DATA_BLOCK "IMAC_MOTOR3_I/O"
TITLE =
AUTHOR : Hottendo
FAMILY : IMAC
VERSION : 0.1


  STRUCT
   MOTOR3_001_ACOM : WORD ;	//MOTOR3 - Instance 001 : 'AUTO' Mode  Command Interface
   MOTOR3_001_STAT : WORD ;	//                        'AUTO' Mode  Status Interface
   MOTOR3_001_OSSTAT : WORD ;	//                        OS Status Word
   MOTOR3_001_OSALARM : WORD ;	//                        OS Alarm Word
   MOTOR3_001_OSCOM : WORD ;	//                        OS Command Interface
   MOTOR3_002_ACOM : WORD ;	//MOTOR3 - Instance 002 : 'AUTO' Mode  Command Interface
   MOTOR3_002_STAT : WORD ;	//                        'AUTO' Mode  Status Interface
   MOTOR3_002_OSSTAT : WORD ;	//                        OS Status Word
   MOTOR3_002_OSALARM : WORD ;	//                        OS Alarm Word
   MOTOR3_002_OSCOM : WORD ;	//                        OS Command Interface
   MOTOR3_003_ACOM : WORD ;	//MOTOR3 - Instance 003 : 'AUTO' Mode  Command Interface
   MOTOR3_003_STAT : WORD ;	//                        'AUTO' Mode  Status Interface
   MOTOR3_003_OSSTAT : WORD ;	//                        OS Status Word
   MOTOR3_003_OSALARM : WORD ;	//                        OS Alarm Word
   MOTOR3_003_OSCOM : WORD ;	//                        OS Command Interface
   MOTOR3_004_ACOM : WORD ;	//MOTOR3 - Instance 004 : 'AUTO' Mode  Command Interface
   MOTOR3_004_STAT : WORD ;	//                        'AUTO' Mode  Status Interface
   MOTOR3_004_OSSTAT : WORD ;	//                        OS Status Word
   MOTOR3_004_OSALARM : WORD ;	//                        OS Alarm Word
   MOTOR3_004_OSCOM : WORD ;	//                        OS Command Interface
   MOTOR3_005_ACOM : WORD ;	//MOTOR3 - Instance 005 : 'AUTO' Mode  Command Interface
   MOTOR3_005_STAT : WORD ;	//                        'AUTO' Mode  Status Interface
   MOTOR3_005_OSSTAT : WORD ;	//                        OS Status Word
   MOTOR3_005_OSALARM : WORD ;	//                        OS Alarm Word
   MOTOR3_005_OSCOM : WORD ;	//                        OS Command Interface
   MOTOR3_006_ACOM : WORD ;	//MOTOR3 - Instance 006 : 'AUTO' Mode  Command Interface
   MOTOR3_006_STAT : WORD ;	//                        'AUTO' Mode  Status Interface
   MOTOR3_006_OSSTAT : WORD ;	//                        OS Status Word
   MOTOR3_006_OSALARM : WORD ;	//                        OS Alarm Word
   MOTOR3_006_OSCOM : WORD ;	//                        OS Command Interface
   MOTOR3_007_ACOM : WORD ;	//MOTOR3 - Instance 007 : 'AUTO' Mode  Command Interface
   MOTOR3_007_STAT : WORD ;	//                        'AUTO' Mode  Status Interface
   MOTOR3_007_OSSTAT : WORD ;	//                        OS Status Word
   MOTOR3_007_OSALARM : WORD ;	//                        OS Alarm Word
   MOTOR3_007_OSCOM : WORD ;	//                        OS Command Interface
   MOTOR3_008_ACOM : WORD ;	//MOTOR3 - Instance 008 : 'AUTO' Mode  Command Interface
   MOTOR3_008_STAT : WORD ;	//                        'AUTO' Mode  Status Interface
   MOTOR3_008_OSSTAT : WORD ;	//                        OS Status Word
   MOTOR3_008_OSALARM : WORD ;	//                        OS Alarm Word
   MOTOR3_008_OSCOM : WORD ;	//                        OS Command Interface
   MOTOR3_009_ACOM : WORD ;	//MOTOR3 - Instance 009 : 'AUTO' Mode  Command Interface
   MOTOR3_009_STAT : WORD ;	//                        'AUTO' Mode  Status Interface
   MOTOR3_009_OSSTAT : WORD ;	//                        OS Status Word
   MOTOR3_009_OSALARM : WORD ;	//                        OS Alarm Word
   MOTOR3_009_OSCOM : WORD ;	//                        OS Command Interface
   MOTOR3_010_ACOM : WORD ;	//MOTOR3 - Instance 010 : 'AUTO' Mode  Command Interface
   MOTOR3_010_STAT : WORD ;	//                        'AUTO' Mode  Status Interface
   MOTOR3_010_OSSTAT : WORD ;	//                        OS Status Word
   MOTOR3_010_OSALARM : WORD ;	//                        OS Alarm Word
   MOTOR3_010_OSCOM : WORD ;	//                        OS Command Interface
   MOTOR3_011_ACOM : WORD ;	//MOTOR3 - Instance 011 : 'AUTO' Mode  Command Interface
   MOTOR3_011_STAT : WORD ;	//                        'AUTO' Mode  Status Interface
   MOTOR3_011_OSSTAT : WORD ;	//                        OS Status Word
   MOTOR3_011_OSALARM : WORD ;	//                        OS Alarm Word
   MOTOR3_011_OSCOM : WORD ;	//                        OS Command Interface
   MOTOR3_012_ACOM : WORD ;	//MOTOR3 - Instance 012 : 'AUTO' Mode  Command Interface
   MOTOR3_012_STAT : WORD ;	//                        'AUTO' Mode  Status Interface
   MOTOR3_012_OSSTAT : WORD ;	//                        OS Status Word
   MOTOR3_012_OSALARM : WORD ;	//                        OS Alarm Word
   MOTOR3_012_OSCOM : WORD ;	//                        OS Command Interface
   MOTOR3_013_ACOM : WORD ;	//MOTOR3 - Instance 013 : 'AUTO' Mode  Command Interface
   MOTOR3_013_STAT : WORD ;	//                        'AUTO' Mode  Status Interface
   MOTOR3_013_OSSTAT : WORD ;	//                        OS Status Word
   MOTOR3_013_OSALARM : WORD ;	//                        OS Alarm Word
   MOTOR3_013_OSCOM : WORD ;	//                        OS Command Interface
   MOTOR3_014_ACOM : WORD ;	//MOTOR3 - Instance 014 : 'AUTO' Mode  Command Interface
   MOTOR3_014_STAT : WORD ;	//                        'AUTO' Mode  Status Interface
   MOTOR3_014_OSSTAT : WORD ;	//                        OS Status Word
   MOTOR3_014_OSALARM : WORD ;	//                        OS Alarm Word
   MOTOR3_014_OSCOM : WORD ;	//                        OS Command Interface
   MOTOR3_015_ACOM : WORD ;	//MOTOR3 - Instance 015 : 'AUTO' Mode  Command Interface
   MOTOR3_015_STAT : WORD ;	//                        'AUTO' Mode  Status Interface
   MOTOR3_015_OSSTAT : WORD ;	//                        OS Status Word
   MOTOR3_015_OSALARM : WORD ;	//                        OS Alarm Word
   MOTOR3_015_OSCOM : WORD ;	//                        OS Command Interface
   MOTOR3_016_ACOM : WORD ;	//MOTOR3 - Instance 016 : 'AUTO' Mode  Command Interface
   MOTOR3_016_STAT : WORD ;	//                        'AUTO' Mode  Status Interface
   MOTOR3_016_OSSTAT : WORD ;	//                        OS Status Word
   MOTOR3_016_OSALARM : WORD ;	//                        OS Alarm Word
   MOTOR3_016_OSCOM : WORD ;	//                        OS Command Interface
   MOTOR3_017_ACOM : WORD ;	//MOTOR3 - Instance 017 : 'AUTO' Mode  Command Interface
   MOTOR3_017_STAT : WORD ;	//                        'AUTO' Mode  Status Interface
   MOTOR3_017_OSSTAT : WORD ;	//                        OS Status Word
   MOTOR3_017_OSALARM : WORD ;	//                        OS Alarm Word
   MOTOR3_017_OSCOM : WORD ;	//                        OS Command Interface
   MOTOR3_018_ACOM : WORD ;	//MOTOR3 - Instance 018 : 'AUTO' Mode  Command Interface
   MOTOR3_018_STAT : WORD ;	//                        'AUTO' Mode  Status Interface
   MOTOR3_018_OSSTAT : WORD ;	//                        OS Status Word
   MOTOR3_018_OSALARM : WORD ;	//                        OS Alarm Word
   MOTOR3_018_OSCOM : WORD ;	//                        OS Command Interface
   MOTOR3_019_ACOM : WORD ;	//MOTOR3 - Instance 019 : 'AUTO' Mode  Command Interface
   MOTOR3_019_STAT : WORD ;	//                        'AUTO' Mode  Status Interface
   MOTOR3_019_OSSTAT : WORD ;	//                        OS Status Word
   MOTOR3_019_OSALARM : WORD ;	//                        OS Alarm Word
   MOTOR3_019_OSCOM : WORD ;	//                        OS Command Interface
   MOTOR3_020_ACOM : WORD ;	//MOTOR3 - Instance 020 : 'AUTO' Mode  Command Interface
   MOTOR3_020_STAT : WORD ;	//                        'AUTO' Mode  Status Interface
   MOTOR3_020_OSSTAT : WORD ;	//                        OS Status Word
   MOTOR3_020_OSALARM : WORD ;	//                        OS Alarm Word
   MOTOR3_020_OSCOM : WORD ;	//                        OS Command Interface
   MOTOR3_021_ACOM : WORD ;	//MOTOR3 - Instance 021 : 'AUTO' Mode  Command Interface
   MOTOR3_021_STAT : WORD ;	//                        'AUTO' Mode  Status Interface
   MOTOR3_021_OSSTAT : WORD ;	//                        OS Status Word
   MOTOR3_021_OSALARM : WORD ;	//                        OS Alarm Word
   MOTOR3_021_OSCOM : WORD ;	//                        OS Command Interface
   MOTOR3_022_ACOM : WORD ;	//MOTOR3 - Instance 022 : 'AUTO' Mode  Command Interface
   MOTOR3_022_STAT : WORD ;	//                        'AUTO' Mode  Status Interface
   MOTOR3_022_OSSTAT : WORD ;	//                        OS Status Word
   MOTOR3_022_OSALARM : WORD ;	//                        OS Alarm Word
   MOTOR3_022_OSCOM : WORD ;	//                        OS Command Interface
   MOTOR3_023_ACOM : WORD ;	//MOTOR3 - Instance 023 : 'AUTO' Mode  Command Interface
   MOTOR3_023_STAT : WORD ;	//                        'AUTO' Mode  Status Interface
   MOTOR3_023_OSSTAT : WORD ;	//                        OS Status Word
   MOTOR3_023_OSALARM : WORD ;	//                        OS Alarm Word
   MOTOR3_023_OSCOM : WORD ;	//                        OS Command Interface
   MOTOR3_024_ACOM : WORD ;	//MOTOR3 - Instance 024 : 'AUTO' Mode  Command Interface
   MOTOR3_024_STAT : WORD ;	//                        'AUTO' Mode  Status Interface
   MOTOR3_024_OSSTAT : WORD ;	//                        OS Status Word
   MOTOR3_024_OSALARM : WORD ;	//                        OS Alarm Word
   MOTOR3_024_OSCOM : WORD ;	//                        OS Command Interface
   MOTOR3_025_ACOM : WORD ;	//MOTOR3 - Instance 025 : 'AUTO' Mode  Command Interface
   MOTOR3_025_STAT : WORD ;	//                        'AUTO' Mode  Status Interface
   MOTOR3_025_OSSTAT : WORD ;	//                        OS Status Word
   MOTOR3_025_OSALARM : WORD ;	//                        OS Alarm Word
   MOTOR3_025_OSCOM : WORD ;	//                        OS Command Interface
  END_STRUCT ;
BEGIN
   MOTOR3_001_ACOM := W#16#0;
   MOTOR3_001_STAT := W#16#0;
   MOTOR3_001_OSSTAT := W#16#0;
   MOTOR3_001_OSALARM := W#16#0;
   MOTOR3_001_OSCOM := W#16#0;
   MOTOR3_002_ACOM := W#16#0;
   MOTOR3_002_STAT := W#16#0;
   MOTOR3_002_OSSTAT := W#16#0;
   MOTOR3_002_OSALARM := W#16#0;
   MOTOR3_002_OSCOM := W#16#0;
   MOTOR3_003_ACOM := W#16#0;
   MOTOR3_003_STAT := W#16#0;
   MOTOR3_003_OSSTAT := W#16#0;
   MOTOR3_003_OSALARM := W#16#0;
   MOTOR3_003_OSCOM := W#16#0;
   MOTOR3_004_ACOM := W#16#0;
   MOTOR3_004_STAT := W#16#0;
   MOTOR3_004_OSSTAT := W#16#0;
   MOTOR3_004_OSALARM := W#16#0;
   MOTOR3_004_OSCOM := W#16#0;
   MOTOR3_005_ACOM := W#16#0;
   MOTOR3_005_STAT := W#16#0;
   MOTOR3_005_OSSTAT := W#16#0;
   MOTOR3_005_OSALARM := W#16#0;
   MOTOR3_005_OSCOM := W#16#0;
   MOTOR3_006_ACOM := W#16#0;
   MOTOR3_006_STAT := W#16#0;
   MOTOR3_006_OSSTAT := W#16#0;
   MOTOR3_006_OSALARM := W#16#0;
   MOTOR3_006_OSCOM := W#16#0;
   MOTOR3_007_ACOM := W#16#0;
   MOTOR3_007_STAT := W#16#0;
   MOTOR3_007_OSSTAT := W#16#0;
   MOTOR3_007_OSALARM := W#16#0;
   MOTOR3_007_OSCOM := W#16#0;
   MOTOR3_008_ACOM := W#16#0;
   MOTOR3_008_STAT := W#16#0;
   MOTOR3_008_OSSTAT := W#16#0;
   MOTOR3_008_OSALARM := W#16#0;
   MOTOR3_008_OSCOM := W#16#0;
   MOTOR3_009_ACOM := W#16#0;
   MOTOR3_009_STAT := W#16#0;
   MOTOR3_009_OSSTAT := W#16#0;
   MOTOR3_009_OSALARM := W#16#0;
   MOTOR3_009_OSCOM := W#16#0;
   MOTOR3_010_ACOM := W#16#0;
   MOTOR3_010_STAT := W#16#0;
   MOTOR3_010_OSSTAT := W#16#0;
   MOTOR3_010_OSALARM := W#16#0;
   MOTOR3_010_OSCOM := W#16#0;
   MOTOR3_011_ACOM := W#16#0;
   MOTOR3_011_STAT := W#16#0;
   MOTOR3_011_OSSTAT := W#16#0;
   MOTOR3_011_OSALARM := W#16#0;
   MOTOR3_011_OSCOM := W#16#0;
   MOTOR3_012_ACOM := W#16#0;
   MOTOR3_012_STAT := W#16#0;
   MOTOR3_012_OSSTAT := W#16#0;
   MOTOR3_012_OSALARM := W#16#0;
   MOTOR3_012_OSCOM := W#16#0;
   MOTOR3_013_ACOM := W#16#0;
   MOTOR3_013_STAT := W#16#0;
   MOTOR3_013_OSSTAT := W#16#0;
   MOTOR3_013_OSALARM := W#16#0;
   MOTOR3_013_OSCOM := W#16#0;
   MOTOR3_014_ACOM := W#16#0;
   MOTOR3_014_STAT := W#16#0;
   MOTOR3_014_OSSTAT := W#16#0;
   MOTOR3_014_OSALARM := W#16#0;
   MOTOR3_014_OSCOM := W#16#0;
   MOTOR3_015_ACOM := W#16#0;
   MOTOR3_015_STAT := W#16#0;
   MOTOR3_015_OSSTAT := W#16#0;
   MOTOR3_015_OSALARM := W#16#0;
   MOTOR3_015_OSCOM := W#16#0;
   MOTOR3_016_ACOM := W#16#0;
   MOTOR3_016_STAT := W#16#0;
   MOTOR3_016_OSSTAT := W#16#0;
   MOTOR3_016_OSALARM := W#16#0;
   MOTOR3_016_OSCOM := W#16#0;
   MOTOR3_017_ACOM := W#16#0;
   MOTOR3_017_STAT := W#16#0;
   MOTOR3_017_OSSTAT := W#16#0;
   MOTOR3_017_OSALARM := W#16#0;
   MOTOR3_017_OSCOM := W#16#0;
   MOTOR3_018_ACOM := W#16#0;
   MOTOR3_018_STAT := W#16#0;
   MOTOR3_018_OSSTAT := W#16#0;
   MOTOR3_018_OSALARM := W#16#0;
   MOTOR3_018_OSCOM := W#16#0;
   MOTOR3_019_ACOM := W#16#0;
   MOTOR3_019_STAT := W#16#0;
   MOTOR3_019_OSSTAT := W#16#0;
   MOTOR3_019_OSALARM := W#16#0;
   MOTOR3_019_OSCOM := W#16#0;
   MOTOR3_020_ACOM := W#16#0;
   MOTOR3_020_STAT := W#16#0;
   MOTOR3_020_OSSTAT := W#16#0;
   MOTOR3_020_OSALARM := W#16#0;
   MOTOR3_020_OSCOM := W#16#0;
   MOTOR3_021_ACOM := W#16#0;
   MOTOR3_021_STAT := W#16#0;
   MOTOR3_021_OSSTAT := W#16#0;
   MOTOR3_021_OSALARM := W#16#0;
   MOTOR3_021_OSCOM := W#16#0;
   MOTOR3_022_ACOM := W#16#0;
   MOTOR3_022_STAT := W#16#0;
   MOTOR3_022_OSSTAT := W#16#0;
   MOTOR3_022_OSALARM := W#16#0;
   MOTOR3_022_OSCOM := W#16#0;
   MOTOR3_023_ACOM := W#16#0;
   MOTOR3_023_STAT := W#16#0;
   MOTOR3_023_OSSTAT := W#16#0;
   MOTOR3_023_OSALARM := W#16#0;
   MOTOR3_023_OSCOM := W#16#0;
   MOTOR3_024_ACOM := W#16#0;
   MOTOR3_024_STAT := W#16#0;
   MOTOR3_024_OSSTAT := W#16#0;
   MOTOR3_024_OSALARM := W#16#0;
   MOTOR3_024_OSCOM := W#16#0;
   MOTOR3_025_ACOM := W#16#0;
   MOTOR3_025_STAT := W#16#0;
   MOTOR3_025_OSSTAT := W#16#0;
   MOTOR3_025_OSALARM := W#16#0;
   MOTOR3_025_OSCOM := W#16#0;
END_DATA_BLOCK

